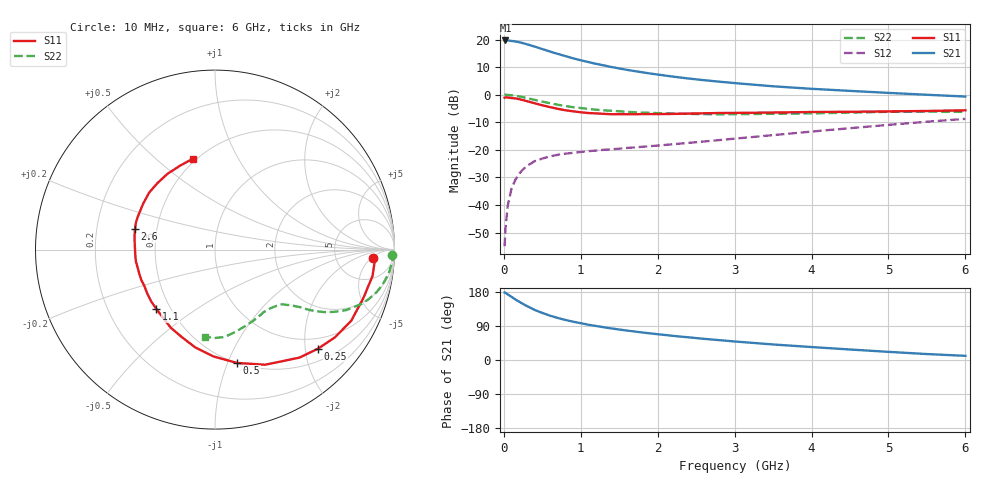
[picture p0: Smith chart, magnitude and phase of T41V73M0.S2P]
! Infineon Technologies  Discrete & RF Semiconductors
! BFR182T
! Si NPN RF Bipolar Junction Transistor in SC75
! VCE = 1.75 V  IC = 3 mA
! Common Emitter S-Parameters:  October  1999
# GHz  S  MA  R  50
!  f  S11  S21  S12  S22
! GHz  MAG  ANG  MAG  ANG  MAG  ANG  MAG  ANG
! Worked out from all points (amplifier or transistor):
!   36 points, 10 MHz to 6 GHz, reference 50 ohm
!   highest |S21| = 19.7 dB at 20 MHz (marker M1)
!   |S21| within 3 dB of that: start of sweep to 487.2 MHz
!   unconditionally stable (mu >= 1): 1.672 GHz to 4.231 GHz
!   at 250 MHz: K = 0.20, MSG = 22.9 dB, |S12| = -27.1 dB
!   at 1.4 GHz: K = 0.91, MSG = 14.9 dB, |S12| = -19.8 dB
!   at 6 GHz: K = 0.84, MSG = 4.0 dB, |S12| = -8.8 dB
!   lowest NFmin = 1.10 dB at 450 MHz
!   S11 on the Smith chart (normalised r, x): 10 MHz: 14, -6; 250 MHz: 0.75, -2.27; 500 MHz: 0.50, -1.08; 1.1 GHz: 0.42, -0.35; 2.6 GHz: 0.37, +0.11; 6 GHz: 0.48, +0.67
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0.01  0.8819 -2.9  9.568 178.1  0.0018 84.7  0.9868 -1.6
0.02  0.8951 -2.3  9.609 177.6  0.0036 92.1  0.9983 -1.6
0.05  0.8899 -9.5  9.587 173.1  0.0097 88.1  0.9896 -4.0
0.1  0.8696 -18.1  9.41 166.8  0.0199 80.7  0.9768 -7.9
0.15  0.8563 -27.6  9.219 159.9  0.0289 74.2  0.9556 -11.5
0.2  0.8282 -36.1  8.935 153.7  0.0372 72.0  0.9309 -14.8
0.25  0.7962 -43.9  8.578 147.8  0.0442 67.3  0.9004 -17.8
0.3  0.7639 -52.0  8.197 142.3  0.0513 64.1  0.87 -20.4
0.4  0.6995 -66.5  7.449 132.2  0.0623 58.0  0.8058 -24.7
0.5  0.6429 -79.1  6.713 124.2  0.0696 53.9  0.7491 -27.6
0.6  0.5951 -90.9  6.049 117.0  0.0763 50.4  0.7005 -29.8
0.7  0.5559 -101.4  5.49 111.0  0.0814 48.5  0.6579 -31.4
0.8  0.5223 -110.5  5.006 105.7  0.0854 46.9  0.6238 -32.6
0.9  0.5002 -119.5  4.565 101.1  0.0883 45.7  0.5939 -33.5
1.1  0.4646 -134.7  3.899 93.0  0.095 45.1  0.5521 -35.0
1.5  0.444 -157.7  2.991 80.4  0.1052 46.6  0.5008 -37.9
2.2  0.4484 175.9  2.125 63.7  0.1266 51.6  0.4563 -44.6
2.6  0.4604 165.5  1.833 55.9  0.1418 54.1  0.4445 -49.6
3.5  0.4753 147.3  1.42 41.0  0.1852 57.9  0.45 -61.7
4.5  0.49 130.9  1.172 27.7  0.2473 57.8  0.4731 -76.4
5.5  0.5068 112.4  0.997 15.7  0.3235 54.2  0.4928 -90.3
6  0.5216 103.5  0.925 11.0  0.365 51.0  0.489 -96.4
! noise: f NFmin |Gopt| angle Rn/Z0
0.45  1.1  0.37  30  0.33
0.9  1.2  0.35  61  0.26
1.8  1.85  0.27  133  0.2
